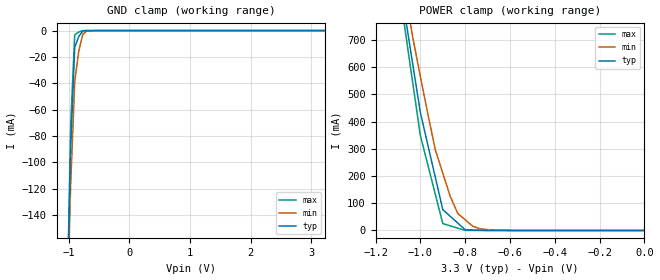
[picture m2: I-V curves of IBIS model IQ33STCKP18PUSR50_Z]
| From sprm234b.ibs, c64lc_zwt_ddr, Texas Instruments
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[Model]   IQ33STCKP18PUSR50_Z
Model_type   Input
Polarity   Non-Inverting
Vinl =  0.8V
Vinh =  2V
C_comp   0.7641276p   0.7005841p   0.8387284p
[Model Spec]
Vinl   0.8V   0.8V   0.8V
Vinh   2V   2V   2V
[Temperature Range]   25   125   -40
[Voltage Range]   3.3   3.14   3.47
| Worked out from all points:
|   GND clamp passes 1 mA (typ) near -0.78 V on its own axis
|   POWER clamp passes 1 mA (typ) near -0.73 V on its own axis
[POWER_clamp]
|   voltage   I(typ)   I(min)   I(max)
-3.3V     15.05A     13.64A     16.17A
-1.067V   781.1mA    866.5mA    727.5mA
-1.033V   606.9mA    705.8mA    537.9mA
-1V       432.7mA    564.8mA    348.3mA
-933.3mV  195.3mA    296.2mA    133mA
-900mV    76.68mA    210.6mA    25.31mA
-866.7mV  52.04mA    125.1mA    16.97mA
-833.3mV  27.39mA    62.68mA    8.616mA
-800mV    2.74mA     39.29mA    267.3uA
-766.7mV  1.853mA    15.91mA    185.4uA
-733.3mV  966.1uA    5.942mA    103.4uA
-11.55fV  95.71nA    92.62nA    222.9nA
[GND_clamp]
|   voltage   I(typ)   I(min)   I(max)
-3.3V     -17.3A     -15.65A    -18.51A
-1.033V   -224.6mA   -230.5mA   -227.5mA
-966.7mV  -89.37mA   -116.8mA   -72.18mA
-900mV    -12.6mA    -38.83mA   -3.274mA
-833.3mV  -4.5mA     -15.57mA   -1.123mA
-766.7mV  -308.1uA   -2.769mA   -32.66uA
-700mV    -20.68uA   -432.9uA   -3.34uA
3.233V    94.11nA    98.66nA    210.4nA
